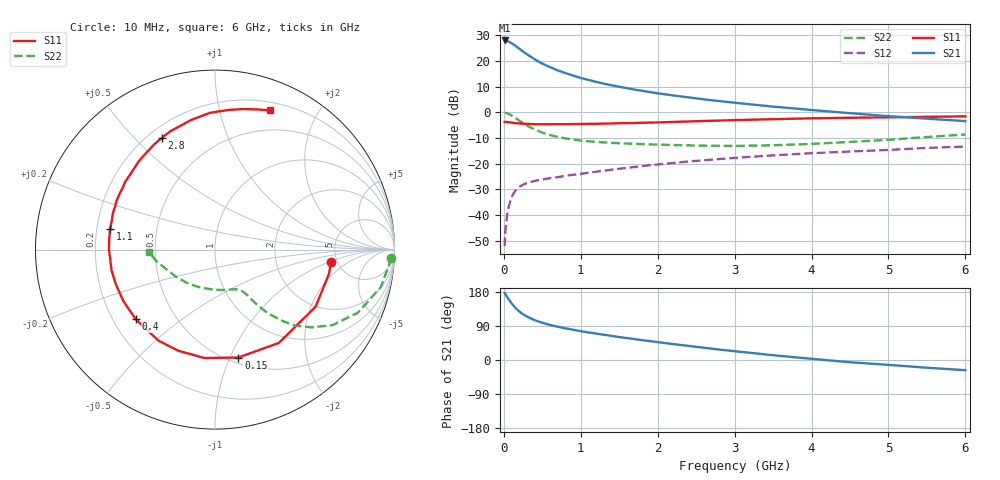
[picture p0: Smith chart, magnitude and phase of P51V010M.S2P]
! SIEMENS Small Signal Semiconductors
! BFP183
! Si NPN RF Bipolar Junction Transistor in SOT143
! VCE = 1 V  IC = 10 mA
! Common Emitter S-Parameters:  March  1996
# GHz  S  MA  R  50
!  f  S11  S21  S12  S22
! GHz  MAG  ANG  MAG  ANG  MAG  ANG  MAG  ANG
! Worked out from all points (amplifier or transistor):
!   36 points, 10 MHz to 6 GHz, reference 50 ohm
!   highest |S21| = 27.9 dB at 10 MHz (marker M1)
!   |S21| within 3 dB of that: start of sweep to 192.1 MHz
!   unconditionally stable (mu >= 1): 1.026 GHz to end of sweep
!   at 250 MHz: K = 0.35, MSG = 25.9 dB, |S12| = -28.2 dB
!   at 1.4 GHz: K = 1.13, MAG = 14.3 dB, |S12| = -22.3 dB
!   at 6 GHz: K = 1.01, MAG = 4.4 dB, |S12| = -13.3 dB
!   S11 on the Smith chart (normalised r, x): 10 MHz: 4.46, -1.03; 150 MHz: 0.56, -1.08; 400 MHz: 0.29, -0.35; 1.1 GHz: 0.26, +0.09; 2.8 GHz: 0.25, +0.60; 6 GHz: 0.28, +1.43
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0.01  0.6501 -5.9  24.89 177.0  0.0025 82.1  0.9791 -2.6
0.02  0.6493 -12.0  24.88 173.9  0.0051 82.4  0.9726 -5.2
0.05  0.6446 -29.6  24.25 164.0  0.0125 78.6  0.9474 -12.7
0.1  0.6301 -55.6  22.03 149.8  0.0225 65.4  0.8698 -23.9
0.15  0.6152 -77.8  19.6 137.7  0.0301 57.5  0.7784 -32.7
0.2  0.6069 -95.6  17.27 128.3  0.0355 51.5  0.6917 -38.8
0.25  0.5996 -110.0  15.11 120.6  0.039 46.6  0.6164 -43.4
0.3  0.5972 -121.7  13.43 114.7  0.0422 44.4  0.5521 -46.4
0.4  0.5879 -138.7  10.73 105.1  0.0463 40.2  0.4634 -50.2
0.5  0.5856 -150.9  8.819 98.2  0.0497 38.5  0.4029 -52.2
0.6  0.585 -160.6  7.563 92.5  0.0523 38.7  0.3604 -53.3
0.7  0.5879 -168.6  6.505 87.7  0.0548 38.7  0.3314 -54.1
0.9  0.5909 179.8  5.171 79.9  0.061 39.8  0.296 -55.4
1.1  0.5956 168.9  4.258 72.6  0.067 40.6  0.2733 -57.2
1.5  0.6127 153.3  3.139 60.5  0.0798 41.5  0.2497 -62.3
1.8  0.6269 143.0  2.613 52.3  0.09 41.4  0.2406 -67.6
2.2  0.6497 130.9  2.127 42.0  0.1033 40.0  0.2312 -76.4
2.8  0.6899 115.3  1.653 27.5  0.1233 36.6  0.2235 -92.7
3.5  0.7343 100.4  1.29 12.6  0.1454 32.0  0.2283 -114.4
4.5  0.7818 84.4  0.961 -5.9  0.1729 24.1  0.2656 -145.6
5.5  0.8155 73.3  0.752 -20.4  0.2031 17.0  0.3316 -168.5
6  0.8337 68.5  0.674 -26.9  0.2159 12.6  0.3698 -178.3
